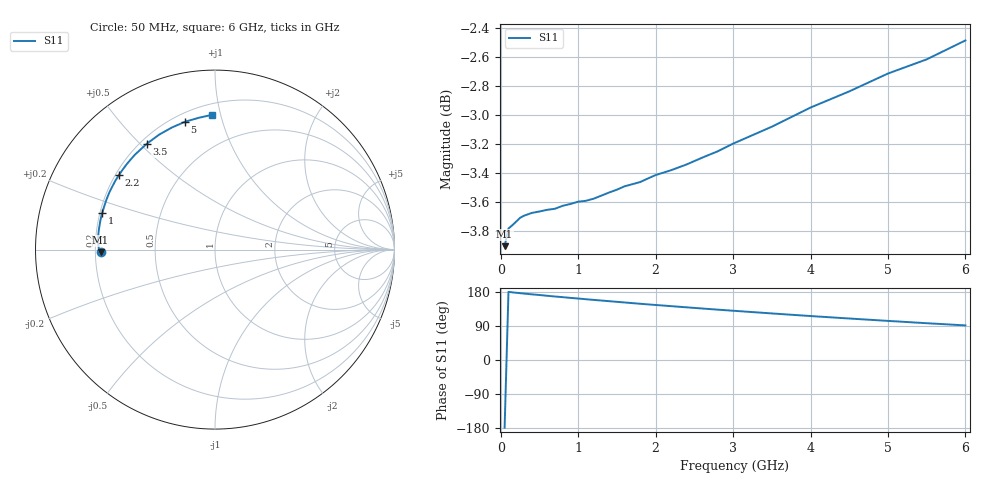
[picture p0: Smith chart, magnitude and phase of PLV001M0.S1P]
! Infineon Technologies  Discrete & RF Semiconductors
! BAR 64-04W /-05W /-06W
! Si PIN Diode in SOT323
! IF = 1 mA
! S-Parameters:  October  2008
# GHz  S  MA  R  50
!  f  S11
! GHz  MAG  ANG
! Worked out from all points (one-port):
!   34 points, 50 MHz to 6 GHz, reference 50 ohm
!   lowest |S11| = -3.9 dB at 50 MHz (marker M1), VSWR 4.53, Z = 11 - j0.581 ohm
!   |S11| at or under -10 dB: nowhere
!   S11 on the Smith chart (normalised r, x): 50 MHz: 0.22, -0.01; 1 GHz: 0.21, +0.15; 2.2 GHz: 0.21, +0.33; 3.5 GHz: 0.23, +0.52; 5 GHz: 0.25, +0.76; 6 GHz: 0.27, +0.94
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0.05  0.6381 -178.6
0.1  0.647 179.8
0.2  0.6506 177.4
0.25  0.6525 176.4
0.3  0.6536 175.3
0.4  0.6551 173.3
0.5  0.6558 171.5
0.6  0.6567 169.5
0.8  0.6588 165.8
0.9  0.6597 163.9
1  0.6609 162.2
1.2  0.6625 158.6
1.4  0.6658 155.2
1.6  0.669 151.8
1.8  0.6713 148.4
1.9  0.6732 146.8
2  0.675 145.2
2.2  0.6776 142.1
2.4  0.6807 139.0
2.6  0.6844 135.9
2.8  0.6878 132.9
3  0.692 130.0
3.5  0.7014 122.9
4  0.7121 116.0
4.5  0.7213 109.5
5  0.7315 103.2
5.5  0.7398 97.1
6  0.751 91.3
